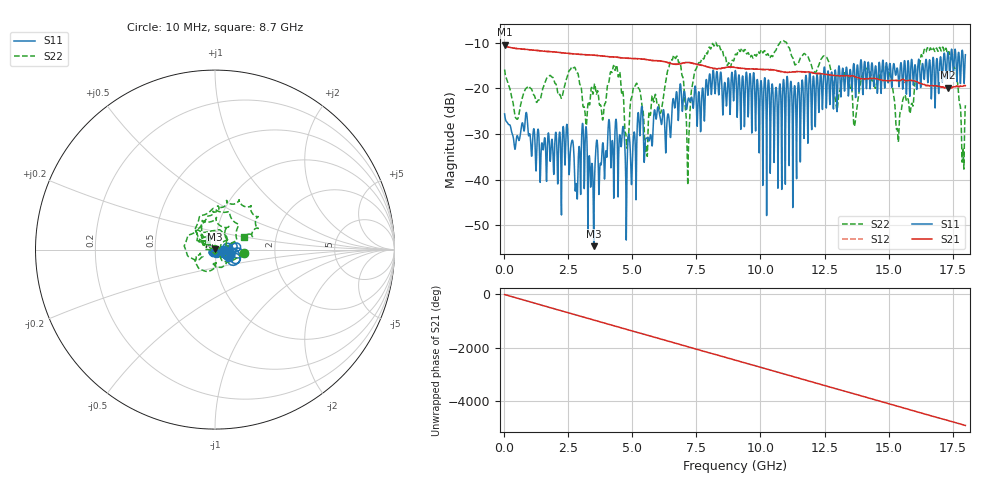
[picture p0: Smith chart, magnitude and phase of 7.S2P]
!Agilent Technologies,E5071C,MY46316741,A.11.02
!Date: Thu Sep 29 15:32:52 2022
!Data & Calibration Information:
!Freq	S11:SOLT2(ON)	S21:SOLT2(ON)	S12:SOLT2(ON)	S22:SOLT2(ON)
!PortZ  Port1:50+j0  Port2:50+j0
!Above PortZ is port z conversion or system Z0 setting when saving the data.
!When reading, reference impedance value at option line is always used.
# Hz S dB R 50
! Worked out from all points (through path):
!   1800 points, 10 MHz to 18 GHz, reference 50 ohm
!   highest |S21| = -10.46 dB at 10 MHz (marker M1); lowest = -19.9 dB at 17.31 GHz (marker M2)
!   group delay of S21, straight-line fit = 756 ps
!   lowest |S11| = -54.6 dB at 3.49 GHz (marker M3), VSWR 1.00, Z = 49.8 + j0.0839 ohm
!   |S11| at or under -10 dB: start of sweep to end of sweep
!   |S22| runs from -41.2 to -9.5 dB; largest |S21 - S12| = 0.013
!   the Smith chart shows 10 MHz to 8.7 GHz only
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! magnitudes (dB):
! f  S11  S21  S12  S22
! 10 MHz  -25.6  -10.5  -10.5  -15.9
! 480 MHz  -30.7  -11.3  -11.3  -26.7
! 3.01 GHz  -32.1  -12.6  -12.6  -20.2
! 3.49 GHz  -54.6  -12.8  -12.8  -20.1
! 4.43 GHz  -40.0  -13.2  -13.2  -16.9
! 4.78 GHz  -41.2  -13.4  -13.4  -33.1
! 5.2 GHz  -26.7  -13.5  -13.5  -19.4
! 5.53 GHz  -30.9  -13.7  -13.7  -32.4
! 6.01 GHz  -24.2  -14.0  -14.0  -23.4
! 6.69 GHz  -22.2  -14.8  -14.8  -13.5
! 7.16 GHz  -22.9  -14.3  -14.4  -41.2
! 7.54 GHz  -26.7  -14.8  -14.8  -15.0
! 9.01 GHz  -16.3  -15.5  -15.5  -12.7
! 12.01 GHz  -25.8  -16.5  -16.6  -15.4
! 13.37 GHz  -15.6  -17.3  -17.3  -17.2
! 13.7 GHz  -20.6  -17.5  -17.4  -27.3
! 14.07 GHz  -14.1  -18.0  -18.1  -15.9
! 15.01 GHz  -17.0  -18.3  -18.4  -16.1
! 15.36 GHz  -16.2  -18.3  -18.3  -30.2
! 16.34 GHz  -14.8  -19.2  -19.2  -13.0
! 17.31 GHz  -12.3  -19.9  -20.0  -12.5
! 18 GHz  -12.7  -19.4  -19.5  -23.7
